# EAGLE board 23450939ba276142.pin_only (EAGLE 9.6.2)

Size 62.23 x 25.4 mm. Coordinates in mm from the lower left corner, seen from the top.
Outline: 3.17,0 arc-90 0,3.17 0,22.23 arc-90 3.17,25.4 59.05,25.4 arc-90 62.23,22.23 62.23,3.17 arc-90 59.05,0 3.17,0
Copper layers (1*16): Top 0.035mm / dielectric 1.5mm / Bottom 0.035mm
Design rules "PCBCart-Standard": minimum track width 8mil, minimum drill 0.4mm, track to track 8mil, track to pad 8mil, pad to pad 8mil, via to via 8mil, smd to smd 8mil, copper to edge 20mil, drill to drill 8mil, minimum pad ring 8mil, minimum via ring 10mil, stop-mask expansion 3mil, vias tented up to drill 20mil, thermal gap 8mil

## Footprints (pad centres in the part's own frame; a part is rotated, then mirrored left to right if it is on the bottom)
0805 = smd 1.3 x 1.5: 1 -0.95,0; 2 0.95,0
E3,5-8 = drill 0.813 pad 1.6: + -1.778,0 | drill 0.813 pad 1.6 octagon: - 1.778,0
FIDUCIAL_1MM = smd 1 x 1: 1 0,0
1X2-3.5MM = drill 1 pad 2.184: 1 1.8,0; 2 -1.7,0
3X04 = drill 1 pad 1.778 square: 1 -3.81,-2.54 | drill 1 pad 1.778: 2 -3.81,0; 3 -3.81,2.54; 4 -1.27,-2.54; 5 -1.27,0; 6 -1.27,2.54; 7 1.27,-2.54; 8 1.27,0; 9 1.27,2.54; 10 3.81,-2.54; 11 3.81,0; 12 3.81,2.54
1X06-CLEANBIG = drill 1.016 pad 1.778 octagon: 1 -6.35,0; 2 -3.81,0; 3 -1.27,0; 4 1.27,0; 5 3.81,0; 6 6.35,0
CHIPLED_0805 = smd 1.2 x 1.2: A 0,-1.05; C 0,1.05
SOT23-WIDE = smd 1 x 1.27: 1 -0.95,-1; 2 0.95,-1; 3 0,1
SOLDERJUMPER_REFLOW_NOPASTE = smd 1.168 x 1.6: 1 -0.762,0; 2 0.762,0
TSSOP28 = smd 0.305 x 0.991: 1 -4.225,-2.918; 2 -3.575,-2.918; 3 -2.925,-2.918; 4 -2.275,-2.918; 5 -1.625,-2.918; 6 -0.975,-2.918; 7 -0.325,-2.918; 8 0.325,-2.918; 9 0.975,-2.918; 10 1.625,-2.918; 11 2.275,-2.918; 12 2.925,-2.918; 13 3.575,-2.918; 14 4.225,-2.918; 15 4.225,2.918; 16 3.575,2.918; 17 2.925,2.918; 18 2.275,2.918; 19 1.625,2.918; 20 0.975,2.918; 21 0.325,2.918; 22 -0.325,2.918; 23 -0.975,2.918; 24 -1.625,2.918; 25 -2.275,2.918; 26 -2.925,2.918; 27 -3.575,2.918; 28 -4.225,2.918
MOUNTINGHOLE_2.5_PLATED = drill 2.5 pad 3.2: P$1 0,0

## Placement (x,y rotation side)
C1  10uF  [0805]  18.99,17.99 180 top
C2  [E3,5-8]  12.32,21.21 180 top
FID1  FIDUCIAL""  [FIDUCIAL_1MM]  45.07,1.36 0 top
FID2  FIDUCIAL""  [FIDUCIAL_1MM]  12.19,23.85 0 top
J1  TERMBLOCK_1X2-3.5MM  [1X2-3.5MM]  31.11,21.59 180 top
JP1  [3X04]  23.49,3.94 180 top
JP2  [3X04]  10.79,3.94 180 top
JP3  [1X06-CLEANBIG]  1.9,12.83 90 top
JP4  [1X06-CLEANBIG]  60.33,12.83 90 top
JP5  [3X04]  51.44,3.94 180 top
JP6  [3X04]  38.73,3.94 180 top
LED1  VCC  [CHIPLED_0805]  22.99,20.07 90 top
Q1  IRLML6401  [SOT23-WIDE]  18.43,23.18 270 top
R1  10K  [0805]  40.89,18.14 90 top
R2  10K  [0805]  43.43,18.14 90 top
R3  10K  [0805]  45.97,18.14 90 top
R4  10K  [0805]  48.51,18.18 90 top
R5  10K  [0805]  51.05,18.18 90 top
R6  10K  [0805]  53.59,18.18 90 top
R7  10K  [0805]  7.11,20.76 90 top
R8  10K  [0805]  6.27,15.94 270 top
R9  10K  [0805]  8.3,15.94 270 top
R10  220  [0805]  18.92,20.07 180 top
R11  220  [0805]  20.57,11.05 90 top
R12  220  [0805]  18.67,11.05 90 top
R13  220  [0805]  16.76,11.05 90 top
R14  220  [0805]  14.86,11.05 90 top
R15  220  [0805]  12.95,11.05 90 top
R16  220  [0805]  11.05,11.05 90 top
R17  220  [0805]  9.14,11.05 90 top
R18  220  [0805]  7.24,11.05 90 top
R19  220  [0805]  55.24,11.05 90 top
R20  220  [0805]  53.34,11.05 90 top
R21  220  [0805]  51.44,11.05 90 top
R22  220  [0805]  49.53,11.05 90 top
R23  220  [0805]  47.62,11.05 90 top
R24  220  [0805]  45.72,11.05 90 top
R25  220  [0805]  43.81,11.05 90 top
R26  220  [0805]  41.91,11.05 90 top
SJ_A0  [SOLDERJUMPER_REFLOW_NOPASTE]  53.59,23.08 270 top
SJ_A1  [SOLDERJUMPER_REFLOW_NOPASTE]  51.05,23.08 270 top
SJ_A2  [SOLDERJUMPER_REFLOW_NOPASTE]  48.51,23.08 270 top
SJ_A3  [SOLDERJUMPER_REFLOW_NOPASTE]  45.97,23.08 270 top
SJ_A4  [SOLDERJUMPER_REFLOW_NOPASTE]  43.43,23.08 270 top
SJ_A5  [SOLDERJUMPER_REFLOW_NOPASTE]  40.89,23.08 270 top
U1  PCA9685  [TSSOP28]  31.11,12.95 270 top
U$47  MOUNTINGHOLE2.5  [MOUNTINGHOLE_2.5_PLATED]  3.17,22.23 0 top
U$48  MOUNTINGHOLE2.5  [MOUNTINGHOLE_2.5_PLATED]  3.17,3.17 0 top
U$49  MOUNTINGHOLE2.5  [MOUNTINGHOLE_2.5_PLATED]  59.05,22.23 0 top
U$50  MOUNTINGHOLE2.5  [MOUNTINGHOLE_2.5_PLATED]  59.05,3.17 0 top
U$51  [ADAFRUIT_5MM]  35.31,9.27 0 top

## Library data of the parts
C1 FID1 FID2 J1 JP1 JP2 JP5 JP6 LED1 Q1 R1-R26 SJ_A0 SJ_A1-SJ_A5 U1 U$47-U$51 = microbuilder
C2 JP3 JP4 = adafruit

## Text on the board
tPlace: adafruit! | POWER | V+ | GND | 1+ | A5 | A4 | A3 | A2 | A1 | A0 | +RW | GND | GND | C2 | OE | OE | PCA9685 | I2C Address | SCL | SCL | 16 x 12-bit PWM | (Open=0/Closed=1) | SDA | SDA | VCC | VCC | 0 | 1 | 2 | 3 | 4 | 5 | 6 | 7 | 8 | 9 | 10 | 11 | 12 | 13 | 14 | 15 | V+ | V+ | PWM | V+ | GND
bPlace: PCA9685 16-Channel 12-Bit PWM Driver | Use V+ for servo supply | 3-5V | VCC: | Terminal block is | 3-5V | Logic: | reverse polarity | 6V Max | V+: | protected. Side breakout | pins are not! | 40-1000Hz | Freq.:
